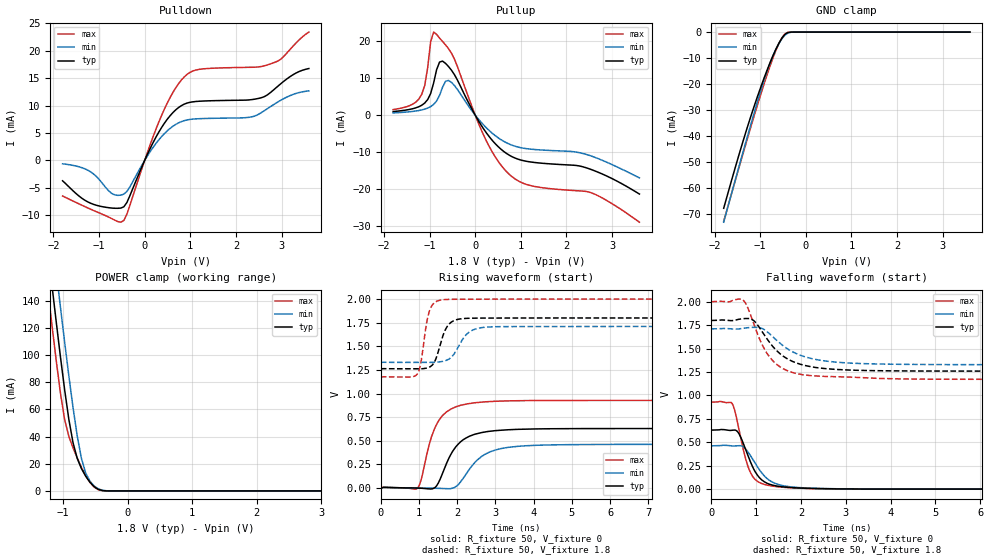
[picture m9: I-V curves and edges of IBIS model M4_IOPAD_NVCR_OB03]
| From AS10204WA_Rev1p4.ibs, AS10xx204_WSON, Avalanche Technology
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[Model] M4_IOPAD_NVCR_OB03
Model_type I/O
Enable   Active-High
Vinl  =  0.54
Vinh  =  1.26
Vmeas =  0.9
Cref  =  30e-12
| Capacitance  typ   min   max
C_comp   3.869840e-12   3.575244e-12   4.208825e-12
| Variables   typ   min   max
[GND Clamp Reference]   0   0   0
[POWER Clamp Reference]   1.8   1.71   2
[Pulldown Reference]   0   0   0
[Pullup Reference]   1.8   1.71   2
[Temperature Range]   25   105   -40
[Voltage Range]   1.8   1.71   2
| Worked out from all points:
|   slope of the pulldown table from 0 to 0.27 V, typ, clamps not added: 59.1 ohm
|   slope of the pullup table from 0 to 0.27 V, typ, clamps not added: 51.8 ohm
|   GND clamp passes 1 mA (typ) near -0.46 V on its own axis
|   POWER clamp passes 1 mA (typ) near -0.44 V on its own axis
|   falling waveform, R_fixture 50, V_fixture 0: 20-80 % time 366ps typ, 445ps min, 295ps max; typ from 0.63 V to 0 V
|   falling waveform, R_fixture 50, V_fixture 1.8: 20-80 % time 674ps typ, 792ps min, 550ps max; typ from 1.8 V to 1.26 V
|   rising waveform, R_fixture 50, V_fixture 0: 20-80 % time 546ps typ, 651ps min, 453ps max; typ from 0 V to 0.63 V
|   rising waveform, R_fixture 50, V_fixture 1.8: 20-80 % time 270ps typ, 374ps min, 191ps max; typ from 1.26 V to 1.8 V
[GND Clamp]
| Voltage   I(typ)   I(min)   I(max)
-1.8V     -67.84mA   -73.19mA   -72.81mA
-1.499V   -49.26mA   -53.93mA   -54.28mA
-1.303V   -37.87mA   -41.64mA   -42.4mA
-1.108V   -27.29mA   -29.68mA   -30.84mA
-912.4mV  -17.6mA    -18.46mA   -19.84mA
-782.1mV  -11.7mA    -11.87mA   -13.01mA
-651.7mV  -6.447mA   -6.494mA   -6.896mA
-521.4mV  -2.255mA   -2.526mA   -2.141mA
-456.2mV  -849.3uA   -1.156mA   -679.4uA
-391mV    -172uA     -356.5uA   -88.88uA
-260.7mV  -2.088uA   -12.98uA   -254.3nA
3.6V      0A         0A         0A
[POWER Clamp]
| Voltage   I(typ)   I(min)   I(max)
-1.8V     419.8mA    456.6mA    390.9mA
-1.238V   178mA      215.7mA    148.4mA
-1.173V   151mA      188.6mA    121.7mA
-1.108V   124.5mA    161.8mA    96mA
-1.043V   98.85mA    135.4mA    72.14mA
-977.6mV  74.56mA    109.6mA    52.56mA
-912.4mV  52.76mA    84.78mA    40.16mA
-847.2mV  35.48mA    61.36mA    31.71mA
-716.9mV  16.42mA    23.91mA    17.31mA
-651.7mV  10.9mA     13.27mA    11.28mA
-456.2mV  1.168mA    1.554mA    921.1uA
3.6V      0A         0A         0A
[Pulldown]
| Voltage   I(typ)   I(min)   I(max)
-1.8V     -3.719mA   -623.4uA   -6.494mA
-1.173V   -7.854mA   -2.154mA   -8.947mA
-716.9mV  -8.695mA   -6.054mA   -10.64mA
-456.2mV  -8.455mA   -6.146mA   -10.94mA
310.3mV   5.166mA    3.752mA    7.006mA
620.7mV   8.732mA    6.235mA    12.41mA
869mV     10.26mA    7.253mA    15.24mA
1.241V    10.81mA    7.618mA    16.65mA
2.352V    11.09mA    7.94mA     16.98mA
2.766V    12.42mA    9.843mA    17.62mA
2.972V    13.9mA     10.91mA    18.37mA
3.6V      16.75mA    12.68mA    23.4mA
[Pullup]
| Voltage   I(typ)   I(min)   I(max)
-1.8V     990uA      623.6uA    1.53mA
-1.173V   2.695mA    1.432mA    5.663mA
-1.108V   3.294mA    1.644mA    8.056mA
-977.6mV  5.876mA    2.33mA     19.91mA
-912.4mV  8.737mA    2.923mA    22.54mA
-782.1mV  14.41mA    5.398mA    20.9mA
-586.6mV  13.21mA    9.435mA    18.06mA
248.3mV   -4.86mA    -3.473mA   -7.072mA
744.8mV   -10.83mA   -7.824mA   -16.02mA
1.241V    -12.73mA   -9.238mA   -19.17mA
2.559V    -14.8mA    -11.13mA   -21.11mA
3.6V      -21.38mA   -17.01mA   -29.01mA
[Ramp]
dV/dt_r   0.377998/0.546255n  0.277411/0.65135n  0.556733/0.452538n
dV/dt_f   0.32444/0.673585n  0.229245/0.79195n  0.497041/0.549934n
R_load = 50
[Falling Waveform]
R_fixture = 50
V_fixture = 0
V_fixture_min = 0
V_fixture_max = 0
| Time   V(typ)   V(min)   V(max)
0s        630mV      462.4mV    927.9mV
458.2ps   627.7mV    460.8mV    917.5mV
516.1ps   630.8mV    460.5mV    847mV
621.6ps   586.2mV    464.2mV    623.8mV
770.2ps   415.7mV    425.4mV    313.3mV
912.3ps   246.8mV    327.7mV    141.6mV
1.176ns   80.2mV     143.6mV    51.62mV
1.538ns   27.86mV    44.06mV    22.68mV
3.407ns   1.201mV    1.831mV    785.7uV
21.88ns   163.6nV    517.6nV    177.4nV
[Falling Waveform]
R_fixture = 50
V_fixture = 1.8
V_fixture_min = 1.71
V_fixture_max = 2
| Time   V(typ)   V(min)   V(max)
0s        1.8V       1.71V      2V
701.2ps   1.819V     1.716V     2.019V
792.2ps   1.821V     1.722V     1.957V
959.5ps   1.792V     1.727V     1.745V
1.151ns   1.668V     1.71V      1.524V
1.334ns   1.543V     1.641V     1.389V
1.742ns   1.378V     1.484V     1.255V
2.229ns   1.306V     1.394V     1.211V
4.436ns   1.261V     1.331V     1.175V
21.88ns   1.259V     1.328V     1.172V
[Rising Waveform]
R_fixture = 50
V_fixture = 0
V_fixture_min = 0
V_fixture_max = 0
| Time   V(typ)   V(min)   V(max)
0s        68.52nV    371.4nV    123.7nV
942.1ps   22.7uV     1.056mV    -6.867mV
1.047ns   -1.804mV   912.5uV    76.76mV
1.326ns   -9.352mV   -839.3uV   541.1mV
1.511ns   58.2mV     -3.007mV   711.2mV
1.937ns   423.1mV    8.123mV    855.4mV
2.443ns   567.1mV    262.1mV    902mV
3.133ns   611.7mV    416.7mV    920.3mV
4.398ns   627.5mV    456.3mV    927mV
21.88ns   630mV      462.4mV    927.9mV
[Rising Waveform]
R_fixture = 50
V_fixture = 1.8
V_fixture_min = 1.71
V_fixture_max = 2
| Time   V(typ)   V(min)   V(max)
0s        1.259V     1.328V     1.172V
948.2ps   1.261V     1.329V     1.203V
1.041ns   1.261V     1.329V     1.311V
1.267ns   1.279V     1.329V     1.867V
1.421ns   1.349V     1.331V     1.967V
1.657ns   1.646V     1.344V     1.994V
1.891ns   1.768V     1.405V     1.998V
2.299ns   1.797V     1.646V     1.999V
2.917ns   1.799V     1.706V     1.999V
21.88ns   1.8V       1.71V      2V
